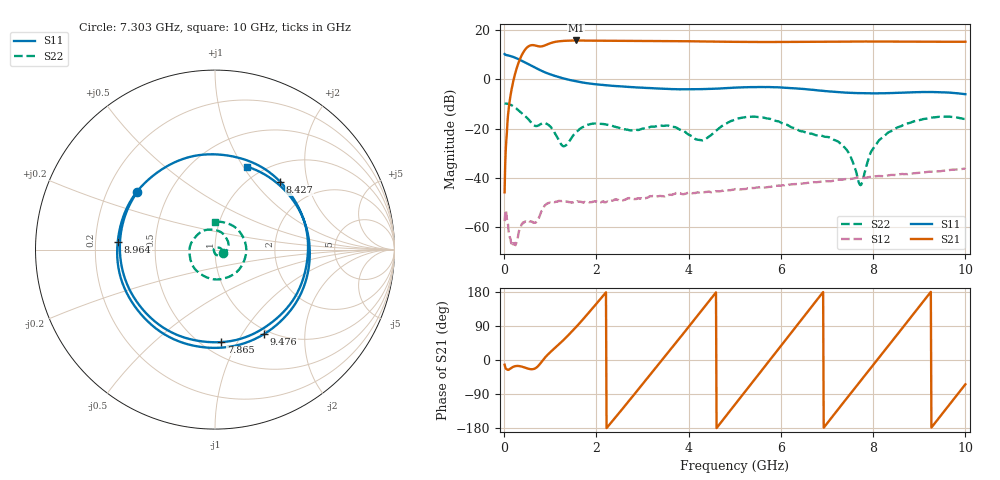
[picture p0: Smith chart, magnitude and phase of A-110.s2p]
! MARKI MICROWAVE INC.
! Email:  info@markimicrowave.com  Phone:  408-778-4200
! Model Number:  A-110  Date:  03/13
! Filename:		A-110.S2P  Version: 1.0
! Description:  2-port S-parameter data for amplifier A-110 measured at -20 dBm input power
! Frequency Measured: 	10 MHz to 10 GHz
! Measurements:		S11, S21, S12, S22
# Hz S  dB  R 50
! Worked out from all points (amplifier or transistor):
!   801 points, 10 MHz to 10 GHz, reference 50 ohm
!   highest |S21| = 15.7 dB at 1.558 GHz (marker M1)
!   |S21| within 3 dB of that: 487.7 MHz to end of sweep
!   unconditionally stable (mu >= 1): 1.387 GHz to end of sweep
!   at 1.671 GHz: K = 6.29, MAG = 21.7 dB, |S12| = -49.8 dB
!   at 5.005 GHz: K = 7.94, MAG = 17.8 dB, |S12| = -44.5 dB
!   at 10 GHz: K = 4.34, MAG = 16.5 dB, |S12| = -36.4 dB
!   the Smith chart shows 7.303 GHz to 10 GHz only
!   S11 on the Smith chart (normalised r, x): 7.303 GHz: 0.33, +0.30; 7.865 GHz: 0.61, -0.86; 8.427 GHz: 1.32, +1.38; 8.964 GHz: 0.30, +0.04; 9.476 GHz: 0.94, -1.25; 10 GHz: 0.85, +1.04
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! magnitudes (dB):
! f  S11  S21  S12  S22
! 10 MHz  10.2  -45.8  -57.5  -9.8
! 84.92 MHz  9.6  -14.4  -59.0  -10.0
! 134.9 MHz  9.4  -7.0  -64.5  -10.3
! 234.8 MHz  8.7  2.0  -66.8  -11.4
! 397.1 MHz  7.3  10.3  -58.6  -14.0
! 684.3 MHz  4.6  13.6  -58.1  -19.0
! 959 MHz  2.2  14.3  -50.2  -18.5
! 1.284 GHz  0.3  15.5  -49.4  -27.2
! 1.558 GHz  -0.8  15.7  -49.6  -21.6
! 1.683 GHz  -1.3  15.6  -49.7  -19.6
! 3.344 GHz  -3.8  15.5  -47.4  -18.8
! 4.293 GHz  -4.0  15.3  -45.7  -24.8
! 5.005 GHz  -3.4  15.1  -44.5  -16.4
! 6.678 GHz  -4.3  15.1  -41.8  -22.1
! 7.303 GHz  -5.4  15.2  -40.7  -26.2
! 7.715 GHz  -5.7  15.3  -39.8  -42.8
! 7.865 GHz  -5.7  15.2  -39.8  -34.5
! 8.339 GHz  -5.7  15.2  -38.9  -21.5
! 8.427 GHz  -5.6  15.2  -38.8  -20.7
! 8.964 GHz  -5.3  15.2  -38.0  -16.8
! 9.476 GHz  -5.3  15.1  -37.2  -15.2
! 10 GHz  -6.1  15.1  -36.4  -16.2
